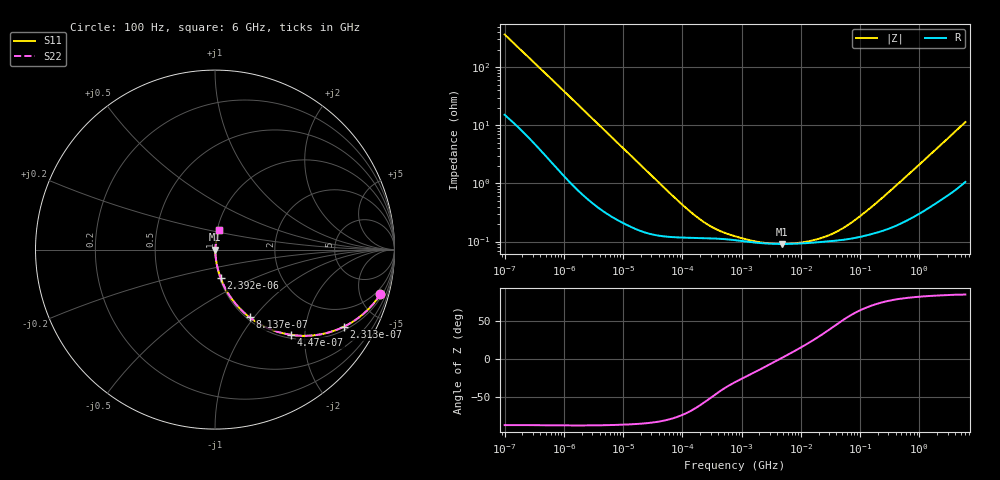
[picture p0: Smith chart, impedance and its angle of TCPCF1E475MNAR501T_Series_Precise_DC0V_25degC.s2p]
! TCPCF1E475MNAR501T Polymer Tantalum Capacitor Sparameter Model
! Model Generated by Samsung Electro-Mechanics
! Samsung Sparameter Version 5.0
! Date : Oct-21-2025
! Products : Polymer Tantalum Capacitor
! Characteristics :
!  Nominal Capacitance = 4.7uF
!  Capacitance Tolerance = +/-20%
!  ESR = 500 mohm max at 100kHz
!  Rated Voltage = 25Vdc
!  Size = 0805(unit:inch), 2012(unit:mm)
!  Length = 2.00+/-0.20mm
!  Width = 1.25+/-0.20mm
!  Thickness = 0.80+/-0.10mm
!  Lineup = Conductive Polymer Type
!  Feature = PCF
!  Measurement Temperature : 25degC.
!  DC bias Value = 0V
!  Frequency : 100Hz ~ 6GHz
! External Node Assignments :
!  1  o---||---o  2
# MHz S RI R 50.0
! Freq.  Real(S11)  Im(S11)  Real(S12)  Im(S12)  Real(S21)  Im(S21)  Real(S22)  Im(S22)
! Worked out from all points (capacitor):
!   300 points, 100 Hz to 6 GHz, reference 50 ohm
!   read as one part in series: C = 4.32 uF near 106.2 Hz
!   lowest |Z| = 91.1 mohm at 4.814 MHz (marker M1)
!   series resonance near 4.523 MHz, so ESL is about 290 pH
!   S11 on the Smith chart (normalised r, x): 100 Hz: 1.30, -7.32; 231.3 Hz: 1.14, -3.24; 447 Hz: 1.07, -1.71; 813.7 Hz: 1.03, -0.95; 2.392 kHz: 1.01, -0.33; 6 GHz: 1.02, +0.23
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0.0001  0.9217 -0.2487  0.0783 0.2487  0.0783 0.2487  0.9217 -0.2487
0.0001520888  0.8457 -0.3407  0.1543 0.3407  0.1543 0.3407  0.8457 -0.3407
0.00023131  0.7168 -0.4301  0.2832 0.4301  0.2832 0.4301  0.7168 -0.4301
0.0004470407  0.4254 -0.4753  0.5746 0.4753  0.5746 0.4753  0.4254 -0.4753
0.0008137405  0.1935 -0.3777  0.8065 0.3777  0.8065 0.3777  0.1935 -0.3777
0.001237608  0.0985 -0.2816  0.9015 0.2816  0.9015 0.2816  0.0985 -0.2816
0.001998454  0.0432 -0.1873  0.9568 0.1873  0.9568 0.1873  0.0432 -0.1873
0.00239186  0.0317 -0.159  0.9683 0.159  0.9683 0.159  0.0317 -0.159
0.007464481  0.00532 -0.0535  0.9947 0.0535  0.9947 0.0535  0.00532 -0.0535
0.03993819  0.00137 -0.0103  0.9986 0.0103  0.9986 0.0103  0.00137 -0.0103
0.2136865  0.00115 -0.00197  0.9988 0.00197  0.9988 0.00197  0.00115 -0.00197
0.3889699  0.00112 -0.00113  0.9989 0.00113  0.9989 0.00113  0.00112 -0.00113
0.7981464  0.00105 -0.000618  0.9989 0.000618  0.9989 0.000618  0.00105 -0.000618
2.081156  0.000942 -0.000233  0.9991 0.000233  0.9991 0.000233  0.000942 -0.000233
4.813922  0.00091 1.78e-05  0.9991 -1.78e-05  0.9991 -1.78e-05  0.00091 1.78e-05
15.95059  0.000957 0.000428  0.999 -0.000428  0.999 -0.000428  0.000957 0.000428
30.82687  0.00101 0.000815  0.999 -0.000815  0.999 -0.000815  0.00101 0.000815
56.11362  0.00109 0.00143  0.9989 -0.00143  0.9989 -0.00143  0.00109 0.00143
115.1423  0.00125 0.00279  0.9988 -0.00279  0.9988 -0.00279  0.00125 0.00279
318.7652  0.00174 0.00716  0.9983 -0.00716  0.9983 -0.00716  0.00174 0.00716
1922.593  0.00601 0.0382  0.994 -0.0382  0.994 -0.0382  0.00601 0.0382
6000  0.0228 0.1097  0.9772 -0.1097  0.9772 -0.1097  0.0228 0.1097
